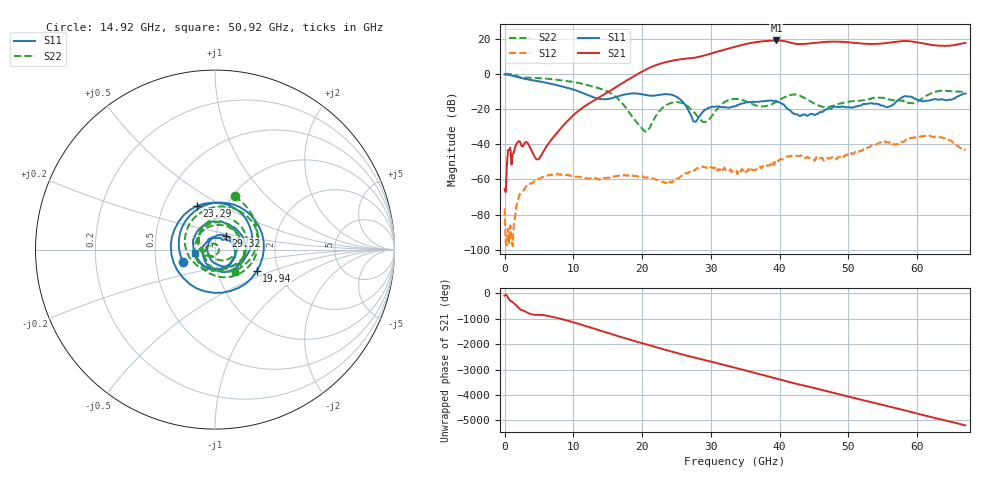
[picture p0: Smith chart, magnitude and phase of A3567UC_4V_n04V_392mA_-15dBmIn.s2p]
! MARKI MICROWAVE INC.
! Date:  4/20/2021
! Model Number:  A-3567UC
! Description:  2-port Small Signal S-parameter data for A-3567UC
! Frequency Range:  10 MHz to 67 GHz
! Port Configuration:  PORT 1: Input
!  PORT 2: Output
! Bias Condition: Vd = +4V, Vg = -0.4V, Id = 392mA
! A-3567UC s2p files are only valid for small signal conditions (below -10 dBm input power)
# Hz S  dB  R 50
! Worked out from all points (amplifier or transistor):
!   401 points, 10 MHz to 67 GHz, reference 50 ohm
!   highest |S21| = 18.9 dB at 39.53 GHz (marker M1)
!   |S21| within 3 dB of that: 34.07 GHz to 63.39 GHz (29.32 GHz wide, 60.2 % of centre)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
!   unconditionally stable (mu >= 1): 172.6 MHz to end of sweep
!   at 11.06 GHz: K = 2892.98, MAG = -18.3 dB, |S12| = -58.8 dB
!   at 33.51 GHz: K = 43.93, MAG = 15.6 dB, |S12| = -54.7 dB
!   at 67 GHz: K = 8.57, MAG = 18.2 dB, |S12| = -43.6 dB
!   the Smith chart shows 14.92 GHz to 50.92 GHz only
!   S11 on the Smith chart (normalised r, x): 14.92 GHz: 0.69, -0.10; 19.94 GHz: 1.54, -0.40; 23.29 GHz: 0.73, +0.38; 29.32 GHz: 1.11, +0.17; 50.92 GHz: 0.80, -0.03
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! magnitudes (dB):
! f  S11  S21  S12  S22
! 10 MHz  -0.4  -65.6  -76.5  0.0
! 679.9 MHz  -0.7  -43.2  -96.3  -0.1
! 1.852 GHz  -1.9  -39.2  -73.5  -1.2
! 4.867 GHz  -4.2  -48.7  -59.5  -2.4
! 11.23 GHz  -10.7  -19.6  -58.9  -5.6
! 14.92 GHz  -14.4  -10.7  -59.1  -10.0
! 19.94 GHz  -11.6  1.1  -58.4  -30.9
! 20.78 GHz  -12.3  2.8  -58.9  -32.5
! 22.45 GHz  -12.0  5.5  -60.6  -21.5
! 23.29 GHz  -11.6  6.5  -61.9  -18.4
! 25.63 GHz  -14.9  8.3  -58.3  -16.5
! 27.64 GHz  -27.2  9.2  -54.9  -22.3
! 29.32 GHz  -20.2  10.7  -53.6  -27.2
! 33.51 GHz  -18.4  15.4  -54.7  -14.2
! 39.53 GHz  -15.5  18.9  -50.2  -15.8
! 42.21 GHz  -22.9  17.1  -46.6  -11.8
! 44.73 GHz  -22.7  17.4  -48.2  -16.3
! 50.92 GHz  -18.9  17.6  -44.5  -15.5
! 55.95 GHz  -18.6  17.7  -39.2  -14.6
! 58.29 GHz  -12.7  18.6  -37.8  -16.2
! 63.15 GHz  -14.7  16.0  -36.0  -9.8
! 67 GHz  -11.2  17.5  -43.6  -10.5
